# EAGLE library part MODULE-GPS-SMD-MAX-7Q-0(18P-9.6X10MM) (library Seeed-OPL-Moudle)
317050009
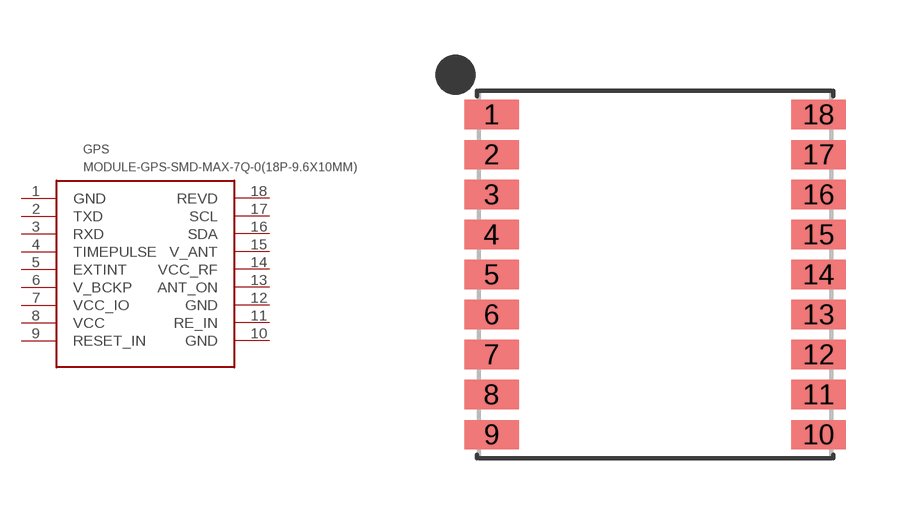
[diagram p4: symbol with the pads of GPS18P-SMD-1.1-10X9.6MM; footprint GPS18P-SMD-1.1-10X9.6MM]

Designator prefix GPS

## MODULE-GPS-SMD-MAX-7Q-0(18P-9.6X10MM) (MPN: MAX-7Q-0; VALUE: MAX-7Q-0(18p-10x9.6mm))  [GPS18P-SMD-1.1-10X9.6MM]
1  GND
2  TXD
3  RXD
4  TIMEPULSE
5  EXTINT
6  V_BCKP
7  VCC_IO
8  VCC
9  RESET_IN
10  GND
11  RE_IN
12  GND
13  ANT_ON
14  VCC_RF
15  V_ANT
16  SDA
17  SCL
18  REVD

## Footprint GPS18P-SMD-1.1-10X9.6MM (pad centres in mm)
smd 1.5 x 0.8: 1 -4.5,4.4; 2 -4.5,3.3; 3 -4.5,2.2; 4 -4.5,1.1; 5 -4.5,0; 6 -4.5,-1.1; 7 -4.5,-2.2; 8 -4.5,-3.3; 9 -4.5,-4.4; 10 4.5,-4.4; 11 4.5,-3.3; 12 4.5,-2.2; 13 4.5,-1.1; 14 4.5,0; 15 4.5,1.1; 16 4.5,2.2; 17 4.5,3.3; 18 4.5,4.4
